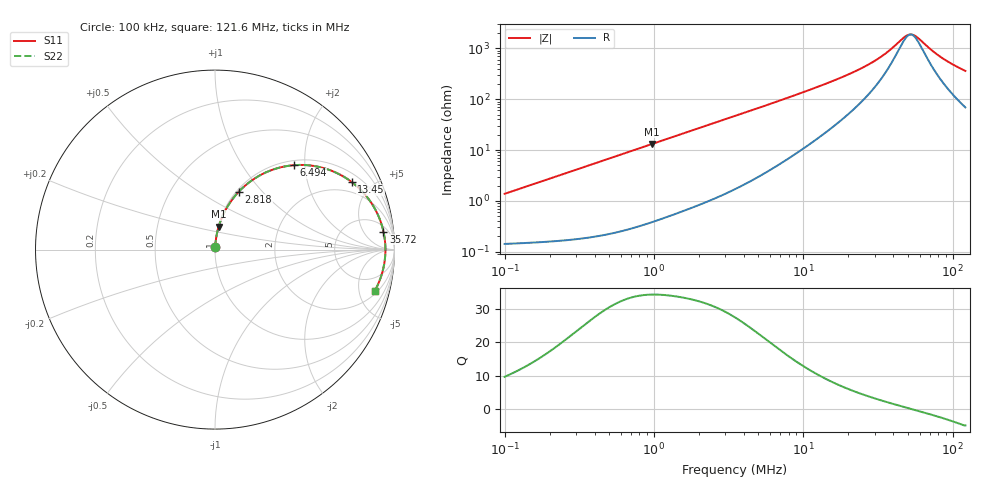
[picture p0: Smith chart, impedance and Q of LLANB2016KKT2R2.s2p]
! LLANB2016KKT2R2  S-PARAMETER MODEL  ( General Type )
! Model Generated by TAIYO YUDEN Corporation (http://www.ty-top.com)
! Version 1.0
! TAIYO YUDEN Control No. 120417NG38SB-FKC
! Copyright(c) 2012 TAIYO YUDEN CO.,LTD. All Rights Reserved.
! Product Description (link to TY-COMPAS)
! https://ds.yuden.co.jp/TYCOMPAS/or/detail?pn=LLANB2016KKT2R2M&u=M
! Products Name : Inductors
! Characteristics :
!  Inductance : 2.2 uH , SRF(min) : -Hz , DC Resistance(max) : 0.16 Ohm
!  Rated Current : Saturation :1500 mA , Temp Rise : 1500 mA (40 degC)
!  Case Size : 2.0 x 1.6 / 0.079 x 0.063 [mm/inch] , Thickness : 1 / 0.039 [mm/inch]
!  (Conditions: Temperature = 25 degC , DC Bias Current/Voltage = 0A / 0V)
! External Node Assignments :
!  1  o---GGG---o  2
! GND o---------o GND
! Frequency Range : 0.1MHz  -  121.638923MHz  [ 402 STEP ]
# MHz S RI R 50
! Freq[MHz].  S11 Real  S11 Imag  S21 Real  S21 Imag  S12 Real  S12 Imag  S22 Real  S22 Imag
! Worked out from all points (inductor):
!   401 points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, 100 kHz to 121.6 MHz, reference 50 ohm
!   read as one part in series: L = 2.18 uH near 103.6 kHz
!   highest Q = 34.4 at 971 kHz (marker M1), where L = 2.15 uH
!   self-resonance near 52.33 MHz
!   S11 on the Smith chart (normalised r, x): 100 kHz: 1.00, +0.03; 2.818 MHz: 1.03, +0.75; 6.494 MHz: 1.09, +1.75; 13.45 MHz: 1.40, +3.79; 35.72 MHz: 8, +15; 121.6 MHz: 2.38, -7.07
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0.1  0.00161 0.0137  0.9984 -0.0137  0.9984 -0.0137  0.00161 0.0137
0.328662  0.00379 0.0444  0.9962 -0.0444  0.9962 -0.0444  0.00379 0.0444
0.971009  0.0205 0.1279  0.9795 -0.1279  0.9795 -0.1279  0.0205 0.1279
1.080188  0.0248 0.1415  0.9752 -0.1415  0.9752 -0.1415  0.0248 0.1415
1.840262  0.0637 0.2294  0.9363 -0.2294  0.9363 -0.2294  0.0637 0.2294
2.81828  0.1327 0.3229  0.8673 -0.3229  0.8673 -0.3229  0.1327 0.3229
3.550168  0.1929 0.3767  0.8071 -0.3767  0.8071 -0.3767  0.1929 0.3767
6.493519  0.4375 0.4701  0.5625 -0.4701  0.5625 -0.4701  0.4375 0.4701
8.475598  0.567 0.4632  0.433 -0.4632  0.433 -0.4632  0.567 0.4632
11.46267  0.7015 0.4152  0.2985 -0.4152  0.2985 -0.4152  0.7015 0.4152
13.44931  0.7612 0.377  0.2388 -0.377  0.2388 -0.377  0.7612 0.377
23.74138  0.8978 0.2145  0.1022 -0.2145  0.1022 -0.2145  0.8978 0.2145
29.38042  0.9236 0.1538  0.0764 -0.1538  0.0764 -0.1538  0.9236 0.1538
35.71886  0.9386 0.1003  0.0614 -0.1003  0.0614 -0.1003  0.9386 0.1003
37.67347  0.9415 0.086  0.0585 -0.086  0.0585 -0.086  0.9415 0.086
48.30734  0.949 0.0208  0.051 -0.0208  0.051 -0.0208  0.949 0.0208
50.95082  0.9494 0.00693  0.0506 -0.00693  0.0506 -0.00693  0.9494 0.00693
53.73896  0.9494 -0.00689  0.0506 0.00689  0.0506 0.00689  0.9494 -0.00689
57.69523  0.9488 -0.0253  0.0512 0.0253  0.0512 0.0253  0.9488 -0.0253
83.77342  0.933 -0.1244  0.067 0.1244  0.067 0.1244  0.933 -0.1244
101.8464  0.9146 -0.179  0.0854 0.179  0.0854 0.179  0.9146 -0.179
121.6389  0.89 -0.2304  0.11 0.2304  0.11 0.2304  0.89 -0.2304
